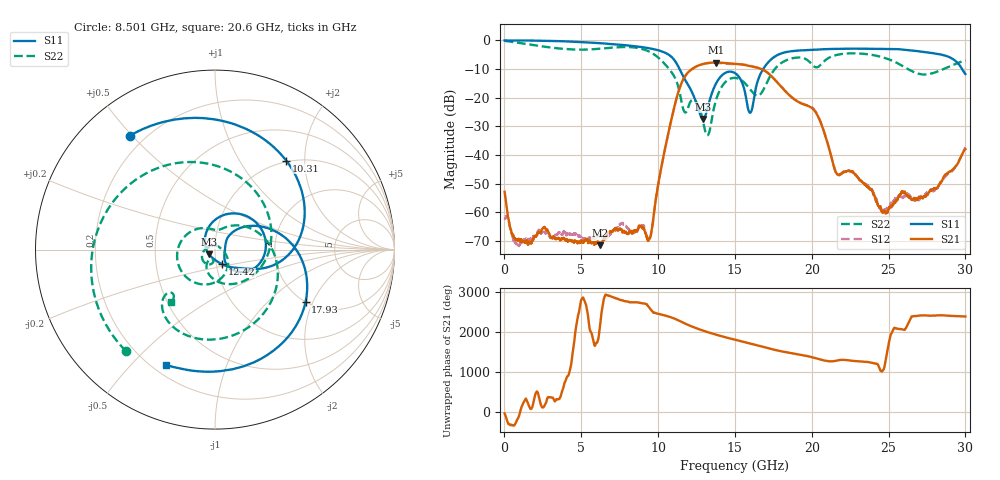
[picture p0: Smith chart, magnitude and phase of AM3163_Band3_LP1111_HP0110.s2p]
!Agilent Technologies,E8364B,MY43040894,A.07.50.67
!Agilent E8364B: A.07.50.67
!Date: Thursday, August 20, 2020 12:15:51
!Correction: S11(Full 2 Port(1,2))
!S21(Full 2 Port(1,2))
!S12(Full 2 Port(1,2))
!S22(Full 2 Port(1,2))
!S2P File: Measurements: S11, S21, S12, S22:
# Hz S  dB  R 50
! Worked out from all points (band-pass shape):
!   3201 points, 10 MHz to 30 GHz, reference 50 ohm
!   highest |S21| = -7.69 dB at 13.78 GHz (marker M1); lowest = -71.4 dB at 6.224 GHz (marker M2)
!   |S21| within 3 dB of the highest: 12.04 GHz to 16.97 GHz (4.936 GHz wide, 34 % of centre)
!   lowest |S11| = -27.4 dB at 12.92 GHz (marker M3), VSWR 1.09, Z = 46.6 - j2.37 ohm
!   |S11| at or under -10 dB: 11.4 GHz to 16.83 GHz (5.434 GHz wide, 38.5 % of centre); 29.79 GHz to end of sweep
!   |S22| runs from -33.1 to -0.1 dB; largest |S21 - S12| = 0.012
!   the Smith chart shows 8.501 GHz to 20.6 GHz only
!   S11 on the Smith chart (normalised r, x): 8.501 GHz: 0.14, +0.49; 10.31 GHz: 0.98, +1.63; 12.42 GHz: 1.07, -0.18; 17.93 GHz: 2.01, -1.76; 20.6 GHz: 0.25, -0.63
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1e7  0.00 -2.0  -52.77 -33.2  -62.51 159.4  -0.13 -5.0
1.247088e9  -0.00 -33.9  -69.96 -117.6  -69.76 -25.1  -1.12 -82.4
2.662241e9  -0.11 -72.2  -65.51 -159.6  -67.32 43.9  -2.22 -163.1
5.014581e9  -0.58 -134.0  -69.84 -56.3  -68.74 128.3  -3.20 72.7
6.223553e9  -0.96 -166.0  -71.39 14.9  -68.10 -22.1  -2.88 5.6
7.544988e9  -1.50 157.0  -65.96 -70.5  -64.06 -70.0  -2.32 -71.2
8.500919e9  -2.02 126.9  -66.27 -131.7  -66.82 -132.7  -2.47 -131.3
9.438106e9  -2.74 92.2  -69.00 91.5  -69.22 -113.0  -3.92 159.0
1.000979e10  -3.42 66.8  -49.94 -57.5  -49.97 -57.9  -5.95 104.4
1.030969e10  -3.94 51.3  -41.35 -85.6  -41.52 -85.4  -7.49 69.0
1.241836e10  -20.74 -63.4  -9.26 -49.0  -9.27 -48.6  -21.00 -141.3
1.292444e10  -27.36 -143.7  -8.21 -118.7  -8.18 -118.4  -28.06 162.8
1.377728e10  -14.94 84.2  -7.69 138.9  -7.79 138.5  -20.69 -39.1
1.5005e10  -11.38 -11.4  -8.15 13.0  -8.23 14.7  -13.05 -147.9
1.599842e10  -25.20 -2.9  -8.90 -83.0  -8.81 -82.5  -17.09 121.0
1.792902e10  -4.70 -29.8  -15.68 90.0  -15.60 90.4  -8.20 -26.6
2.000958e10  -3.29 -98.7  -23.55 -65.7  -23.35 -65.1  -8.34 -137.4
2.060001e10  -3.12 -112.9  -28.84 -129.8  -28.71 -129.8  -8.38 -129.9
2.164966e10  -2.93 -137.7  -46.70 -148.7  -46.55 -152.8  -5.01 -161.9
2.500479e10  -3.00 144.7  -58.59 -85.8  -58.59 121.6  -6.56 67.7
2.740399e10  -4.09 77.2  -54.32 -98.1  -53.61 -110.3  -11.88 -88.0
3e10  -11.70 -27.7  -37.91 -125.8  -37.26 -126.7  -6.98 130.3
